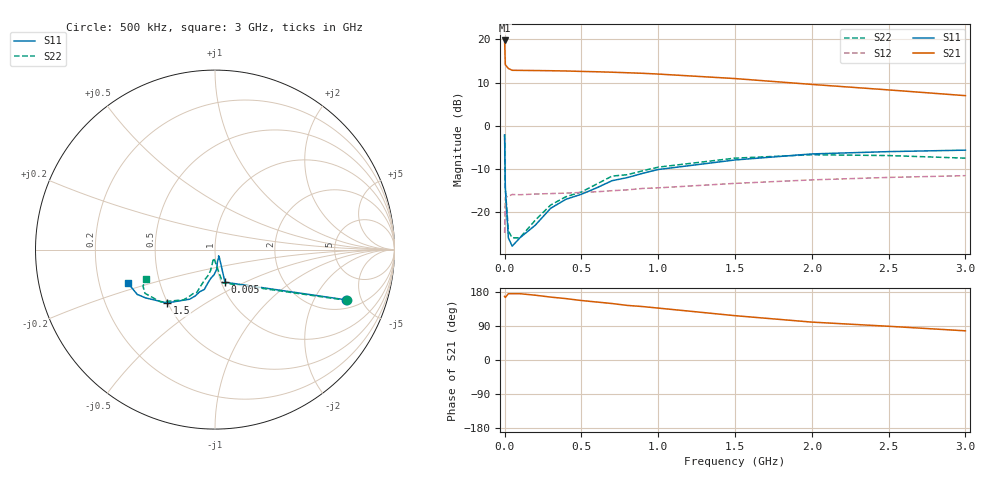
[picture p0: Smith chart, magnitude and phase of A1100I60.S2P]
!  MSA-1100 S AND NOISE PARAMETERS
!  Id=60mA  LAST UPDATED 07-27-92
# ghz s ma r 50
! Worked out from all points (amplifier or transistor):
!   18 points, 500 kHz to 3 GHz, reference 50 ohm
!   highest |S21| = 19.8 dB at 500 kHz (marker M1)
!   |S21| within 3 dB of that: start of sweep to 2.895 MHz
!   unconditionally stable (mu >= 1): 10.18 MHz to 454.4 MHz
!   at 50 MHz: K = 1.06, MAG = 12.9 dB, |S12| = -16.0 dB
!   at 600 MHz: K = 0.96, MSG = 13.9 dB, |S12| = -15.3 dB
!   at 3 GHz: K = 0.67, MSG = 9.3 dB, |S12| = -11.6 dB
!   lowest NFmin = 3.30 dB at 100 MHz
!   S11 on the Smith chart (normalised r, x): 500 kHz: 2.58, -3.68; 5 MHz: 1.04, -0.39; 1.5 GHz: 0.50, -0.35; 3 GHz: 0.33, -0.17
0.0005  0.78 -21.0  9.74 168.0  0.057 50.0  0.79 -21.0
0.005  0.19 -73.0  5.09 165.0  0.147 11.0  0.19 -77.0
0.025  0.05 -61.0  4.61 175.0  0.152 3.0  0.06 -92.0
0.05  0.04 -60.0  4.39 175.0  0.159 3.0  0.05 -102.0
0.1  0.05 -66.0  4.38 175.0  0.158 2.0  0.05 -100.0
0.2  0.07 -79.0  4.36 171.0  0.161 4.0  0.08 -101.0
0.3  0.11 -85.0  4.34 166.0  0.163 6.0  0.12 -102.0
0.4  0.14 -92.0  4.31 162.0  0.165 7.0  0.15 -105.0
0.5  0.16 -98.0  4.26 157.0  0.168 9.0  0.17 -108.0
0.6  0.19 -102.0  4.22 153.0  0.171 11.0  0.21 -111.0
0.7  0.23 -105.0  4.17 149.0  0.176 11.0  0.26 -113.0
0.8  0.25 -110.0  4.11 144.0  0.18 13.0  0.27 -116.0
0.9  0.28 -113.0  4.05 141.0  0.187 12.0  0.3 -119.0
1  0.31 -117.0  3.97 137.0  0.19 14.0  0.33 -122.0
1.5  0.4 -132.0  3.52 117.0  0.214 15.0  0.42 -136.0
2  0.47 -145.0  3.01 100.0  0.235 14.0  0.46 -148.0
2.5  0.5 -150.0  2.6 89.0  0.251 16.0  0.45 -153.0
3  0.52 -159.0  2.23 77.0  0.263 17.0  0.42 -157.0
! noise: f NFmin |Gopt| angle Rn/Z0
0.1  3.3  0.01  104  0.4
0.5  3.5  0.04  122  0.4
1  4  0.08  144  0.39
2  4.6  0.19  174  0.37
